{attribute 'call_after_init'}
FUNCTION_BLOCK FB_DS_IED_LD1_LLN0_DS2 EXTENDS FB_AcsiCommonDataSetClass
VAR
END_VAR

METHOD OnInit : BOOL
VAR
END_VAR
IF NOT DeleteAllMembers() THEN RETURN; END_IF
IF NOT AddMember(ipData:=fbIED.IEDLD1.LEDGGIO1.DPCSO1, eFc:=E_AcsiFc.ST_) THEN RETURN; END_IF
IF NOT AddMember(ipData:=fbIED.IEDLD1.LEDGGIO2.DPCSO1, eFc:=E_AcsiFc.ST_) THEN RETURN; END_IF
IF NOT AddMember(ipData:=fbIED.IEDLD1.LEDGGIO3.DPCSO1, eFc:=E_AcsiFc.ST_) THEN RETURN; END_IF
IF NOT AddMember(ipData:=fbIED.IEDLD1.LEDGGIO4.DPCSO1, eFc:=E_AcsiFc.ST_) THEN RETURN; END_IF
IF NOT AddMember(ipData:=fbIED.IEDLD1.LEDGGIO5.DPCSO1, eFc:=E_AcsiFc.ST_) THEN RETURN; END_IF
IF NOT AddMember(ipData:=fbIED.IEDLD1.LEDGGIO6.DPCSO1, eFc:=E_AcsiFc.ST_) THEN RETURN; END_IF
IF NOT AddMember(ipData:=fbIED.IEDLD1.LEDGGIO7.DPCSO1, eFc:=E_AcsiFc.ST_) THEN RETURN; END_IF
IF NOT AddMember(ipData:=fbIED.IEDLD1.LEDGGIO8.DPCSO1, eFc:=E_AcsiFc.ST_) THEN RETURN; END_IF
OnInit:= TRUE;
END_METHOD

END_FUNCTION_BLOCK
